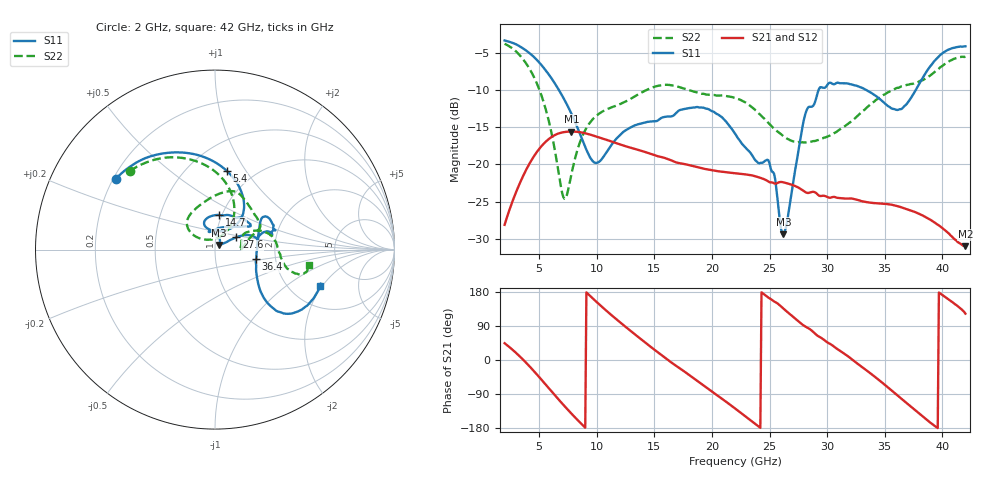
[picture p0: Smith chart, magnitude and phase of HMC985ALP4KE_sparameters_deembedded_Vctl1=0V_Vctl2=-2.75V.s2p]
!s2p File: Measurements: S11, S21, S12, S22
# GHz S dB R 50.0
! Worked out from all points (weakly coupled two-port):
!   401 points, 2 GHz to 42 GHz, reference 50 ohm
!   highest |S21| = -15.58 dB at 7.8 GHz (marker M1); lowest = -31.0 dB at 42 GHz (marker M2)
!   lowest |S11| = -29.4 dB at 26.2 GHz (marker M3), VSWR 1.07, Z = 52.3 + j2.63 ohm
!   |S11| at or under -10 dB: 6.71 GHz to 29.26 GHz (22.55 GHz wide, 125 % of centre); 33.38 GHz to 37.7 GHz (4.313 GHz wide, 12.1 % of centre)
!   |S22| runs from -24.6 to -3.8 dB; largest |S21 - S12| = 0.00069
!   S11 on the Smith chart (normalised r, x): 2 GHz: 0.21, +0.31; 5.4 GHz: 0.75, +0.82; 14.7 GHz: 0.97, +0.39; 27.6 GHz: 1.26, +0.18; 36.4 GHz: 1.58, -0.18; 42 GHz: 2.92, -1.90
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2  -3.36 144.4  -28.09 44.3  -28.07 44.3  -3.80 137.3
3.5  -4.33 118.0  -21.90 4.1  -21.91 4.0  -5.69 105.1
5.4  -7.05 81.7  -17.21 -59.0  -17.22 -59.0  -11.70 65.5
7.1  -11.05 54.8  -15.67 -118.3  -15.70 -118.3  -24.38 90.2
7.8  -13.19 49.7  -15.58 -141.4  -15.56 -141.4  -21.31 138.2
8.7  -16.51 52.8  -15.71 -169.6  -15.72 -169.6  -16.37 145.8
10  -19.78 87.4  -16.27 152.7  -16.25 152.7  -13.42 137.2
14.7  -14.22 83.1  -18.57 34.3  -18.55 34.3  -9.74 80.4
15.4  -13.98 73.9  -18.94 18.2  -18.96 18.1  -9.42 74.7
19.3  -12.40 33.8  -20.56 -67.3  -20.57 -67.3  -10.53 43.5
22  -15.85 52.2  -21.17 -127.8  -21.18 -127.8  -11.07 26.1
25  -19.86 99.2  -22.38 162.7  -22.35 162.7  -14.60 14.8
26.2  -29.36 47.7  -22.39 135.7  -22.42 135.7  -16.20 4.0
27.6  -17.27 30.0  -23.19 99.6  -23.20 99.6  -17.00 -2.7
28.1  -13.25 21.0  -23.70 88.4  -23.73 88.4  -17.05 -1.4
28.7  -12.23 13.0  -23.67 76.6  -23.66 76.5  -16.91 2.5
31  -9.05 23.3  -24.49 26.7  -24.47 26.7  -15.40 26.0
33.3  -9.92 34.2  -25.02 -24.7  -25.01 -24.8  -12.58 26.3
35.4  -12.27 11.9  -25.36 -75.4  -25.34 -75.4  -10.24 17.1
36.4  -12.58 -13.3  -25.72 -100.9  -25.75 -101.0  -9.54 11.0
39.5  -5.83 -43.4  -27.98 -177.5  -27.93 -177.6  -7.36 -15.1
42  -4.15 -18.9  -30.96 122.3  -30.97 122.3  -5.54 -9.4
